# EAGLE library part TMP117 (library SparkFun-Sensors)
Temperature Sensor TMP117x High-Accuracy, Low-Power, Digital Temperature Sensor With SMBus™- and I2C-Compatible Interface
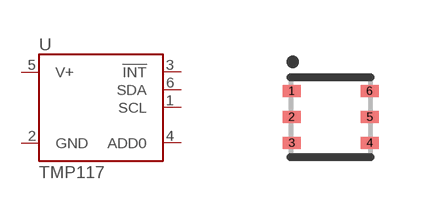
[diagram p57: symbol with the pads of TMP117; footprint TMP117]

Designator prefix U

## TMP117 (PROD_ID: IC-14700)  [TMP117]
1  SCL
2  GND
3  !INT
4  ADD0
5  V+  pwr
6  SDA

## Footprint TMP117 (pad centres in mm)
smd 0.45 x 0.3: 1 -0.975,0.65; 2 -0.975,0; 3 -0.975,-0.65; 4 0.975,-0.65; 5 0.975,0; 6 0.975,0.65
